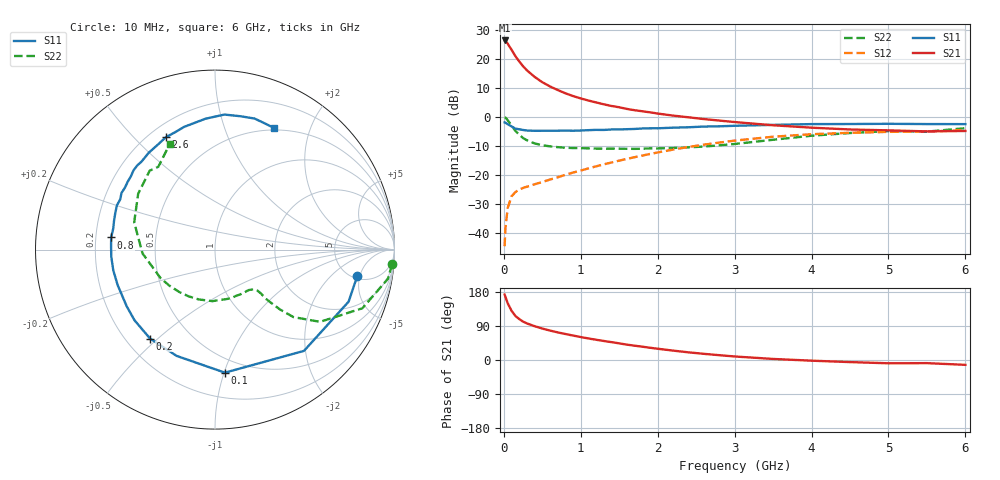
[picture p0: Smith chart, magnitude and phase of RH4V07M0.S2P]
! SIEMENS Small Signal Semiconductors
! BFR106
! Si NPN RF Bipolar Junction Transistor in SOT23
! VCE = 4 V  IC = 7 mA
! Common Emitter S-Parameters:  August  1996
# GHz  S  MA  R  50
!  f  S11  S21  S12  S22
! GHz  MAG  ANG  MAG  ANG  MAG  ANG  MAG  ANG
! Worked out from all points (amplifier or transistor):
!   36 points, 10 MHz to 6 GHz, reference 50 ohm
!   highest |S21| = 26.4 dB at 10 MHz (marker M1)
!   |S21| within 3 dB of that: start of sweep to 94.97 MHz
!   unconditionally stable (mu >= 1): 555.9 MHz to 2.044 GHz; 4.997 GHz to end of sweep
!   at 250 MHz: K = 0.59, MSG = 21.0 dB, |S12| = -24.5 dB
!   at 1.4 GHz: K = 1.12, MAG = 7.7 dB, |S12| = -15.7 dB
!   at 6 GHz: K = 1.02, MAG = -0.9 dB, |S12| = -4.6 dB
!   S11 on the Smith chart (normalised r, x): 10 MHz: 5.42, -4.56; 100 MHz: 0.39, -1.01; 200 MHz: 0.30, -0.47; 800 MHz: 0.26, +0.05; 2.6 GHz: 0.26, +0.62; 6 GHz: 0.48, +1.49
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0.01  0.8064 -10.5  20.93 172.7  0.0059 85.4  0.9901 -4.7
0.02  0.7989 -21.3  20.68 167.1  0.0117 79.4  0.9769 -9.6
0.05  0.7511 -48.7  18.4 149.8  0.0269 66.7  0.8838 -21.7
0.1  0.6878 -85.4  14.46 130.0  0.0427 53.4  0.7106 -34.5
0.15  0.6296 -109.9  11.23 116.2  0.0506 45.3  0.5769 -40.7
0.2  0.6136 -126.1  9.082 108.0  0.0559 42.6  0.4943 -42.6
0.25  0.5969 -138.6  7.519 101.2  0.0597 42.0  0.4329 -43.5
0.3  0.5848 -147.2  6.391 96.6  0.0627 42.9  0.3965 -44.0
0.4  0.5773 -159.9  4.923 89.2  0.069 44.8  0.3502 -43.7
0.5  0.5784 -168.5  3.981 83.0  0.0755 47.9  0.3251 -44.1
0.6  0.5793 -176.2  3.366 77.6  0.0833 50.7  0.3117 -45.5
0.8  0.5825 173.3  2.567 68.6  0.1006 55.5  0.2945 -49.8
0.9  0.579 168.3  2.297 64.5  0.1099 57.1  0.2913 -52.1
1.1  0.5927 159.4  1.922 56.8  0.1298 59.5  0.2874 -59.1
1.6  0.6159 142.2  1.377 40.6  0.1894 61.0  0.2827 -78.9
2.2  0.6539 124.3  1.056 24.8  0.2739 56.7  0.2921 -108.0
2.6  0.6838 113.5  0.921 16.3  0.3328 51.4  0.3089 -130.2
3.5  0.731 94.2  0.72 2.8  0.4566 36.0  0.4045 -177.0
4.5  0.7565 79.1  0.609 -5.5  0.5342 17.6  0.5292 144.0
5  0.7628 73.2  0.588 -8.7  0.5535 9.7  0.5708 129.6
5.5  0.7552 67.7  0.564 -8.3  0.5621 5.8  0.5592 124.4
6  0.7533 64.1  0.574 -12.8  0.5921 -2.0  0.6408 113.1
